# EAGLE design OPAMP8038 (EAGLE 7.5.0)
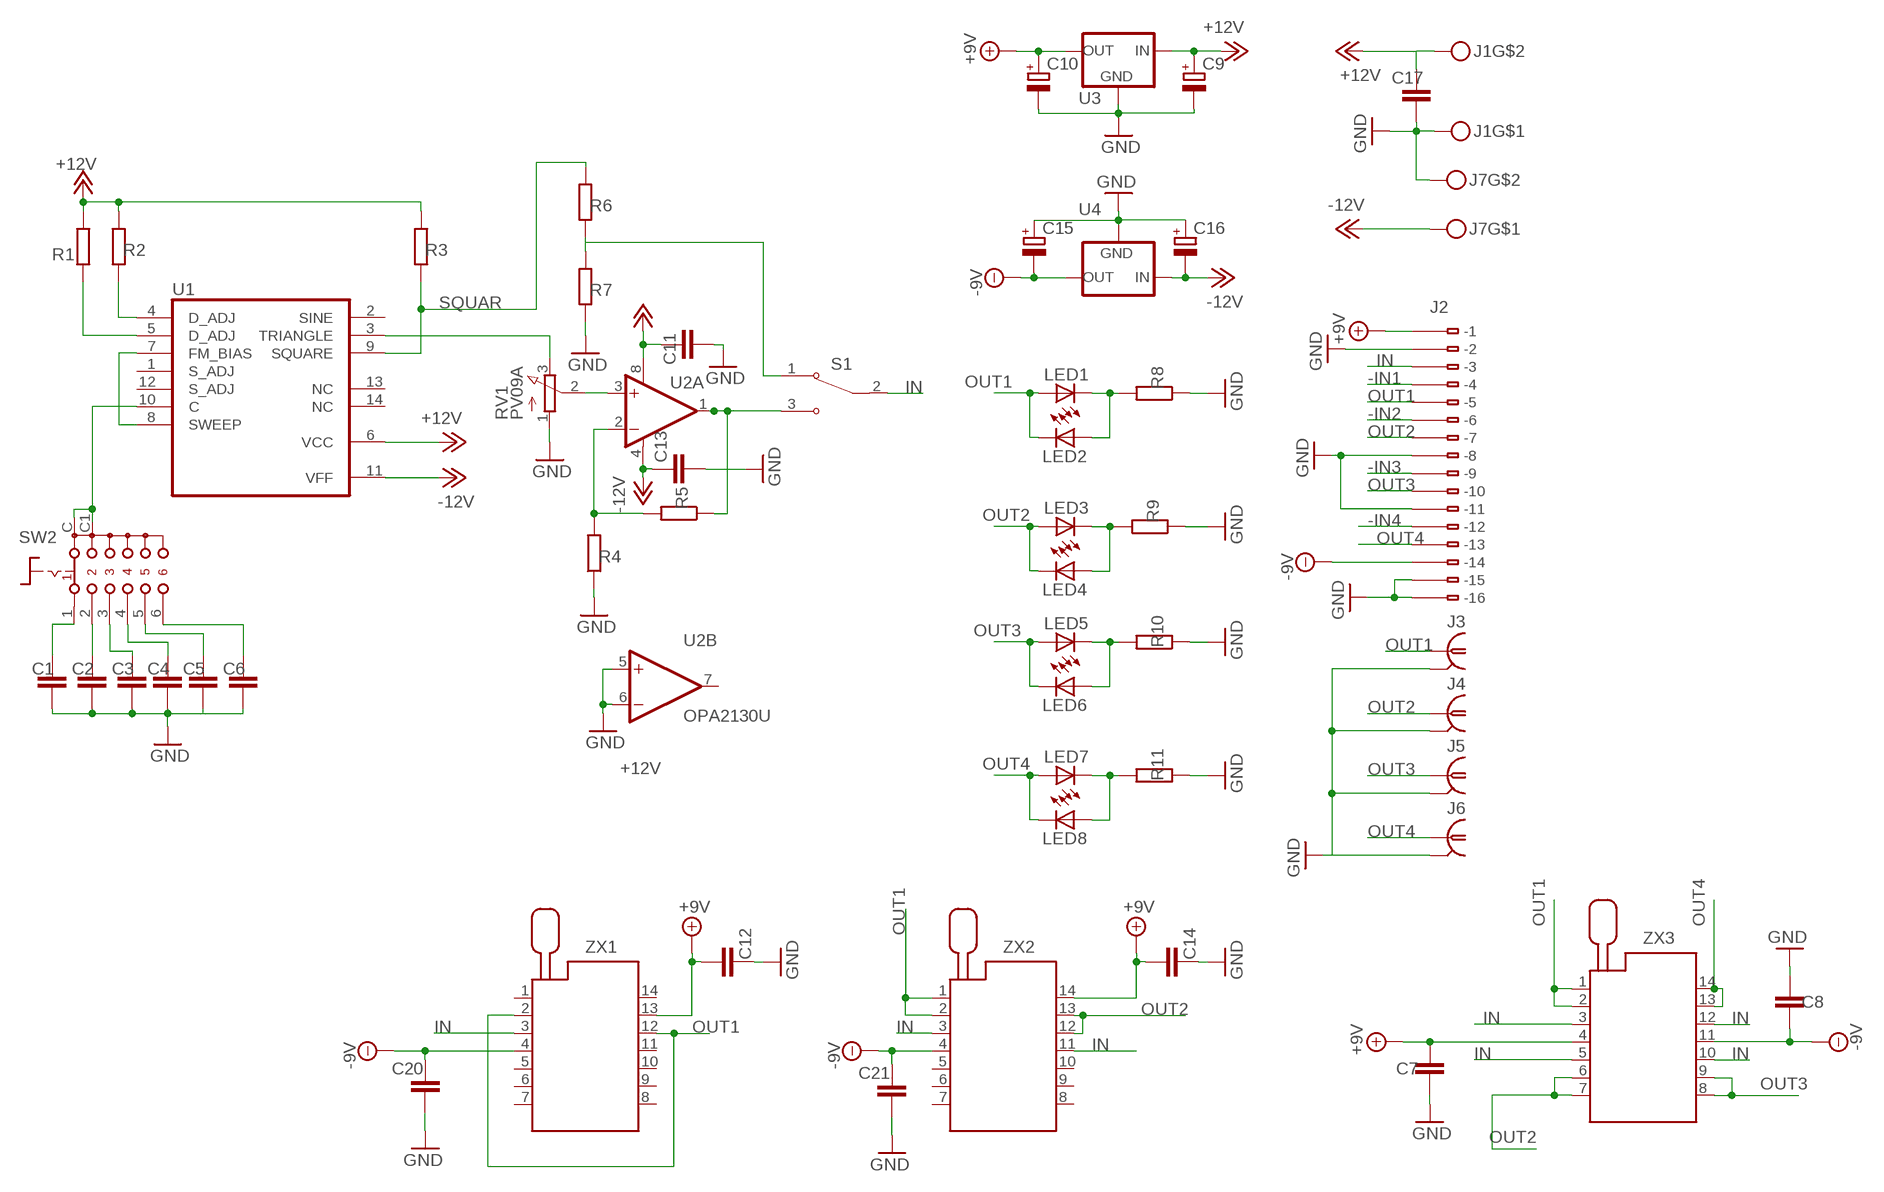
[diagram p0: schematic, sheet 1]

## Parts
C1  C-EUC1206  [C1206]
C2  C-EUC1206  [C1206]
C3  C-EUC1206  [C1206]
C4  C-EUC1206  [C1206]
C5  C-EUC1206  [C1206]
C6  C-EUC1206  [C1206]
C7  C-EUC1206  [C1206]
C8  C-EUC1206  [C1206]
C9  CPOL-EUSMCC  [SMC_C]
C10  CPOL-EUSMCC  [SMC_C]
C11  C-EUC1206  [C1206]
C12  C-EUC1206  [C1206]
C13  C-EUC1206  [C1206]
C14  C-EUC1206  [C1206]
C15  CPOL-EUSMCC  [SMC_C]
C16  CPOL-EUSMCC  [SMC_C]
C17  C-EUC1206  [C1206]
C20  C-EUC1206  [C1206]
C21  C-EUC1206  [C1206]
J1  MKDSN1,5-2-5,08  [MKDSN1,5-2-5,08]
J2  233-116  [233-116]
J3  1-227161-0  [AMP_227161]
J4  1-227161-0  [AMP_227161]
J5  1-227161-0  [AMP_227161]
J6  1-227161-0  [AMP_227161]
J7  MKDSN1,5-2-5,08  [MKDSN1,5-2-5,08]
LED1  LED5MM  [LED5MM]
LED2  LED5MM  [LED5MM]
LED3  LED5MM  [LED5MM]
LED4  LED5MM  [LED5MM]
LED5  LED5MM  [LED5MM]
LED6  LED5MM  [LED5MM]
LED7  LED5MM  [LED5MM]
LED8  LED5MM  [LED5MM]
R1  R-EU_R1206  [R1206]
R2  R-EU_R1206  [R1206]
R3  R-EU_R1206  [R1206]
R4  R-EU_R1206  [R1206]
R5  R-EU_R1206  [R1206]
R6  R-EU_R1206  [R1206]
R7  R-EU_R1206  [R1206]
R8  R-EU_R1206  [R1206]
R9  R-EU_R1206  [R1206]
R10  R-EU_R1206  [R1206]
R11  R-EU_R1206  [R1206]
RV1  PV09A  [PTV09]
S1  100SP1T6B11M1QE  [SW_100SP1T6B11M1QE]
SW2  SS-10-16  [SS-10-16]
U1  XR-8038  [DIL14]
U2  OPA2130U  [SO08]
U3  78XXL  [78XXL]
U4  79XXL  [79XXL]
ZX1  214-3339-00-0602J  [214-3339-00-0602J]
ZX2  214-3339-00-0602J  [214-3339-00-0602J]
ZX3  214-3339-00-0602J  [214-3339-00-0602J]

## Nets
+9V: C7.1 C10.+ C12.2 C14.2 J2.B1(B-1) U3.OUT ZX1.13 ZX2.14 ZX3.4
+12V: C9.+ C11.1 C17.1 J1.2 R1.2 R2.2 R3.2 U1.6(VCC) U2.8(A:V+) U3.IN
-9V: C8.1 C15.- C20.1 C21.1 J2.B14(B-14) U4.OUT ZX1.4 ZX2.4 ZX3.11
-12V: C13.1 C16.- J7.1 U1.11(VFF) U2.4(A:V-) U4.IN
-IN1: J2.B4(B-4)
-IN2: J2.B6(B-6)
-IN3: J2.B9(B-9)
-IN4: J2.B12(B-12)
GND: C1.2 C2.2 C3.2 C4.2 C5.2 C6.2 C7.2 C8.2 C9.- C10.- C11.2 C12.1 C13.2 C14.1 C15.+ C16.+ C17.2 C20.2 C21.2 J1.1 J2.B2(B-2) J2.B8(B-8) J2.B11(B-11) J2.B15(B-15) J2.B16(B-16) J3.2 J4.2 J5.2 J6.2 J7.2 R4.1 R7.1 R8.1 R9.1 R10.1 R11.1 RV1.1(A) U2.5(B:+IN) U2.6(B:-IN) U3.GND U4.GND
IN: J2.B3(B-3) S1.2 ZX1.3 ZX2.3 ZX2.11 ZX3.3 ZX3.5 ZX3.10 ZX3.12
N$1: R6.1 R7.2 S1.1
N$2: C6.1 SW2.6
N$3: R2.1 U1.4(D_ADJ)
N$4: R1.1 U1.5(D_ADJ)
N$5: RV1.2(S) U2.3(A:+IN)
N$6: RV1.3(E) U1.3(TRIANGLE)
N$7: R4.2 R5.2 U2.2(A:-IN)
N$8: R5.1 S1.3 U2.1(A:OUT)
N$9: U1.7(FM_BIAS) U1.8(SWEEP)
N$10: SW2.C SW2.C1 U1.10(C)
N$11: LED1.K(C) LED2.A R8.2
N$12: C1.1 SW2.1
N$13: C2.1 SW2.2
N$14: C3.1 SW2.3
N$15: C4.1 SW2.4
N$16: C5.1 SW2.5
N$18: LED3.K(C) LED4.A R9.2
N$20: LED5.K(C) LED6.A R10.2
N$23: LED7.K(C) LED8.A R11.2
OUT1: J2.B5(B-5) J3.1 LED1.A LED2.K(C) ZX1.2 ZX1.12 ZX2.1 ZX2.2 ZX3.1 ZX3.2
OUT2: J2.B7(B-7) J4.1 LED3.A LED4.K(C) ZX2.12 ZX2.13 ZX3.6 ZX3.7
OUT3: J2.B10(B-10) J5.1 LED5.A LED6.K(C) ZX3.8 ZX3.9
OUT4: J2.B13(B-13) J6.1 LED7.A LED8.K(C) ZX3.13 ZX3.14
SQUAR: R3.1 R6.2 U1.9(SQUARE)
Unconnected: J2.A1(-1) J2.A2(-2) J2.A3(-3) J2.A4(-4) J2.A5(-5) J2.A6(-6) J2.A7(-7) J2.A8(-8) J2.A9(-9) J2.A10(-10) J2.A11(-11) J2.A12(-12) J2.A13(-13) J2.A14(-14) J2.A15(-15) J2.A16(-16) U1.1(S_ADJ) U1.2(SINE) U1.12(S_ADJ) U1.13(NC) U1.14(NC) U2.7(B:OUT) ZX1.1 ZX1.5 ZX1.6 ZX1.7 ZX1.8 ZX1.9 ZX1.10 ZX1.11 ZX1.14 ZX2.5 ZX2.6 ZX2.7 ZX2.8 ZX2.9 ZX2.10

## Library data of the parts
C1-C8 C11-C14 C17 C20 C21 = rcl:C-EU: CAPACITOR, European symbol
C9 C10 C15 C16 = rcl:CPOL-EU: POLARIZED CAPACITOR, European symbol
J1 J7 = con-phoenix-508:MKDSN1,5-2-5,08
J2 = con-wago:233-116: WAGO Cage Clamp; MPN: 233-116; OC_FARNELL: unknown; OC_NEWARK: 28K9054
J3-J6 = con-coax:?227161*: JACK, RIGHT ANGLE, 50 OHM, PCB, BNC; MF: TYCO ELECTRONICS; MPN: 1-227161; OC_FARNELL: unknown; OC_NEWARK: 33B3200
LED1-LED8 = led:LED: LED
R1-R11 = rcl:R-EU_: RESISTOR, European symbol
RV1 = pot:PV09A
S1 = 100SP1T6B11M1QE:100SP1T6B11M1QE: Check availability; AVAILABILITY: Not in stock; CHECK_PRICES: https://www.snapeda.com/parts/100SP1T6B11M1QE/E-Switch/view-part/?ref=eda; DESCRIPTION: Toggle Switches TOGGLE, SPDT , On-On, Panel Mount; MF: E-Switch; MP: 100SP1T6B11M1QE; PACKAGE: None; PRICE: None; SNAPEDA_LINK: https://www.snapeda.com/parts/100SP1T6B11M1QE/E-Switch/view-part/?ref=snap
SW2 = switch:SS-10-16: Rotary Switch, Through Hole, 6 Position, 1 Pole
U1 = exar:XR-8038: Precision WAVEFORM GENERATOR; OC_FARNELL: unknown; OC_NEWARK: unknown
U2 = burr-brown:OPA2130: Operational Amplifier; MF: TEXAS INSTRUMENTS; MPN: OPA2130UA; OC_FARNELL: 1459554; OC_NEWARK: 35C1841
U3 = v-reg:78XXL: VOLTAGE REGULATOR
U4 = v-reg:79XXL: VOLTAGE REGULATOR
ZX1-ZX3 = con-3m:214-3339-00-0602J: Zero Insertion Force Socked Source: http://www.3M.com/ehpd; MF: 3M; MPN: 214-3339-00-0602J; OC_FARNELL: 1247151; OC_NEWARK: 85K7793

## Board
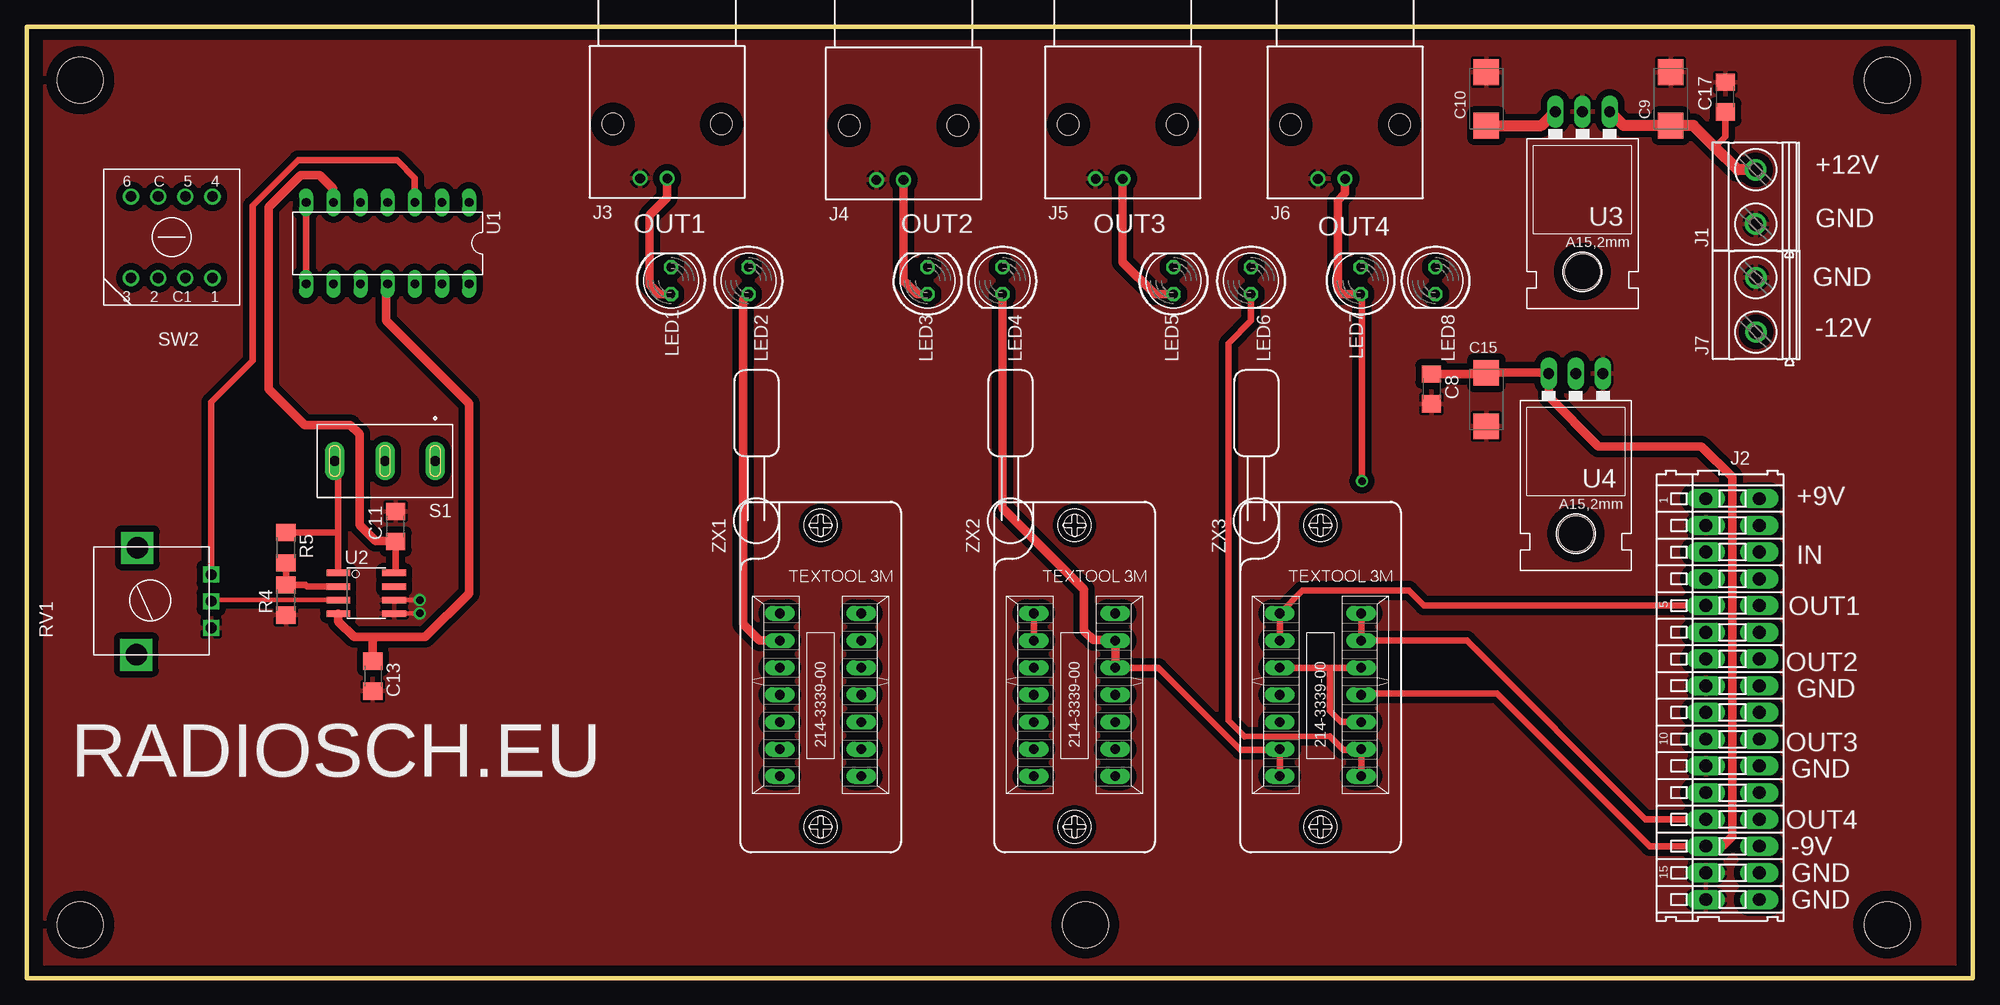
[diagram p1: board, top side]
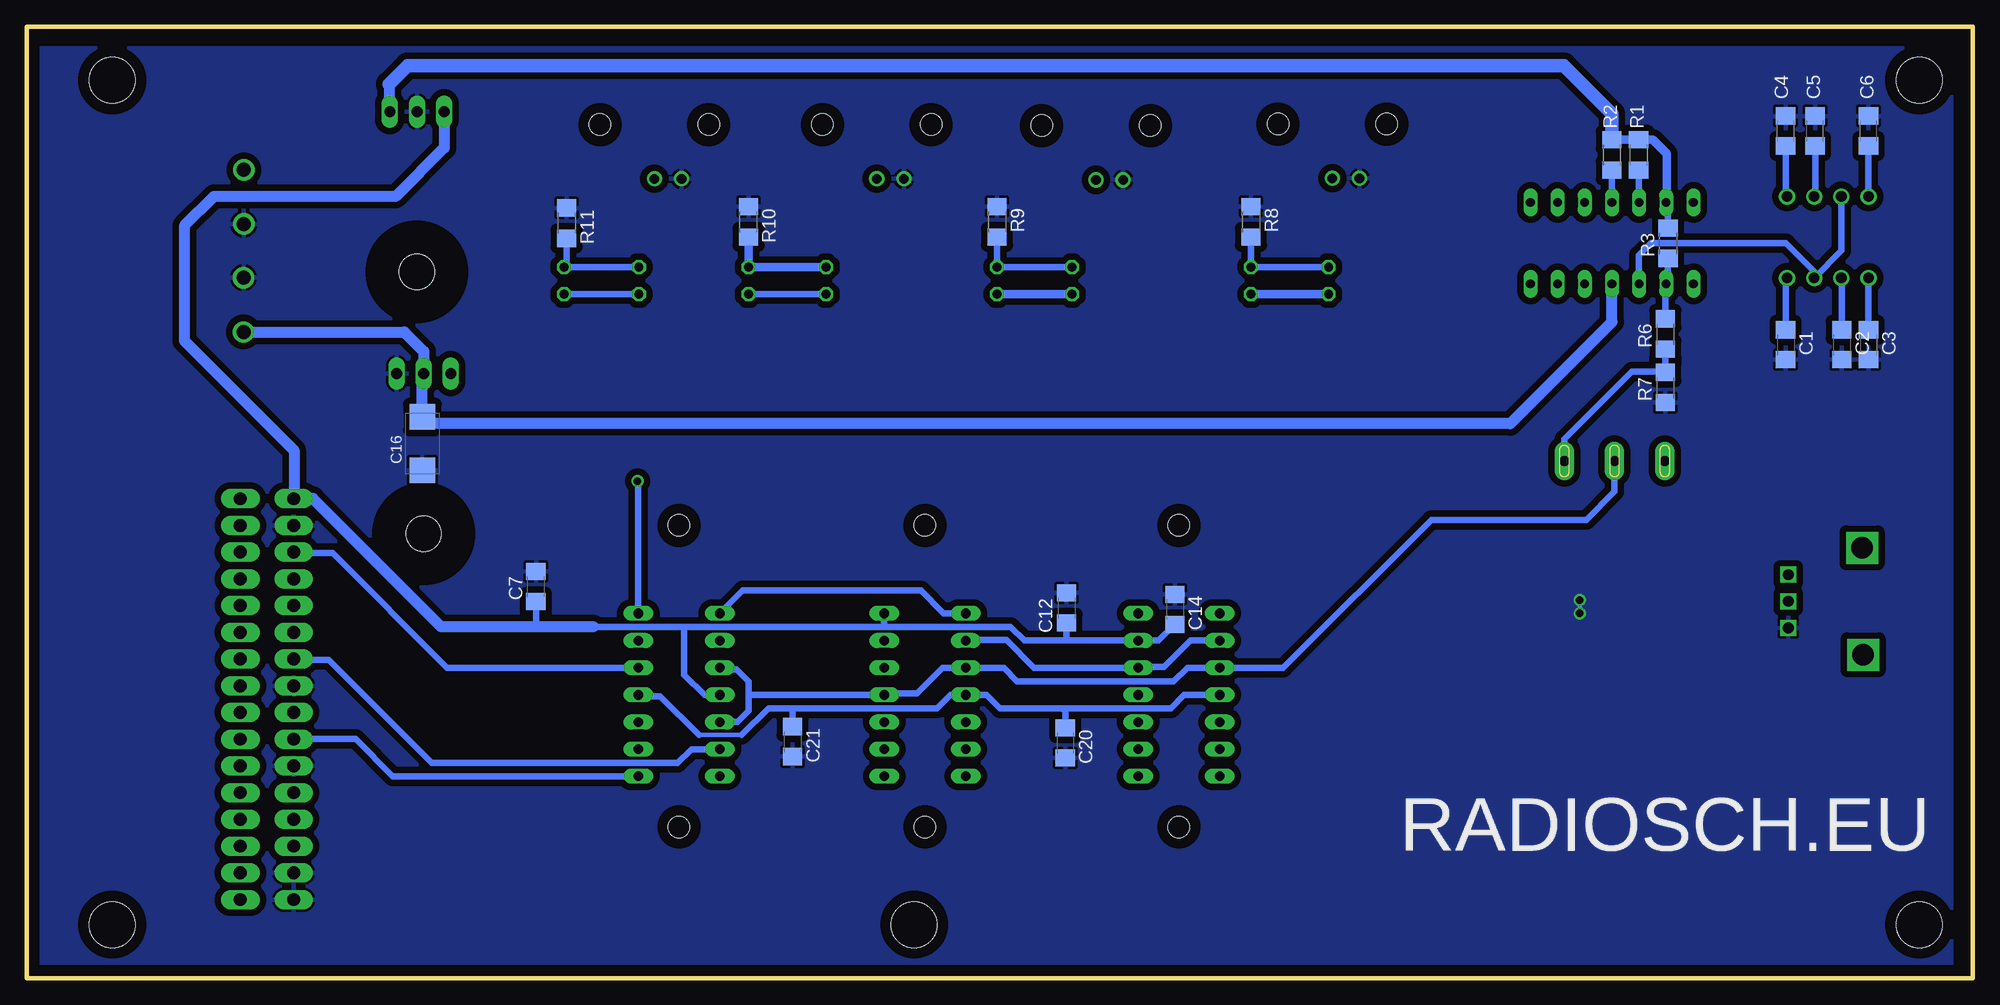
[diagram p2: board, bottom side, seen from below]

Size 182 x 89 mm. Coordinates in mm from the lower left corner, seen from the top.
Outline: 0,0 182,0 182,89 0,89 0,0
Copper layers (1*16): Top 0.035mm / dielectric 1.5mm / Bottom 0.035mm
Design rules "default": minimum track width 10mil, minimum drill 24mil, track to track 8mil, track to pad 8mil, pad to pad 8mil, via to via 8mil, smd to smd 8mil, copper to edge 40mil, drill to drill 8mil, minimum pad ring 10mil, minimum via ring 8mil, stop-mask expansion 4mil, vias tented up to drill 0mil, thermal gap 10mil
Holes 4.3 mm at 5,84 5,5 99,5 174,5 174,84

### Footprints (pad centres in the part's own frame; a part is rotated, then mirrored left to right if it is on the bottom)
C1206 = smd 1.6 x 1.8: 1 -1.4,0; 2 1.4,0
SMC_C = smd 2.4 x 2.4: + -2.5,0; - 2.5,0
MKDSN1,5-2-5,08 = drill 1.3 pad 2: 1 -2.561,0.025; 2 2.519,0.025
233-116 = drill 1.2 long: A1 -18.75,2.5; A2 -16.25,2.5; A3 -13.75,2.5; A4 -11.25,2.5; A5 -8.75,2.5; A6 -6.25,2.5; A7 -3.75,2.5; A8 -1.25,2.5; A9 1.25,2.5; A10 3.75,2.5; A11 6.25,2.5; A12 8.75,2.5; A13 11.25,2.5; A14 13.75,2.5; A15 16.25,2.5; A16 18.75,2.5; B1 -18.75,-2.5; B2 -16.25,-2.5; B3 -13.75,-2.5; B4 -11.25,-2.5; B5 -8.75,-2.5; B6 -6.25,-2.5; B7 -3.75,-2.5; B8 -1.25,-2.5; B9 1.25,-2.5; B10 3.75,-2.5; B11 6.25,-2.5; B12 8.75,-2.5; B13 11.25,-2.5; B14 13.75,-2.5; B15 16.25,-2.5; B16 18.75,-2.5
AMP_227161 = drill 0.9 pad 1.27: 1 0,-5.08; 2 -2.54,-5.08 | hole 2: -5.08,0; 5.08,0
LED5MM = drill 0.813 octagon: A -1.27,0; K 1.27,0
R1206 = smd 1.6 x 1.803: 1 -1.422,0; 2 1.422,0
PTV09 = drill 1 square: 1 -2.5,0; 2 0,0; 3 2.5,0 | drill 2 square: P$4 -5,7; P$5 5,6.9
SW_100SP1T6B11M1QE = drill 0.91 pad 1.81 long: 1 -4.7,0; 2 0,0; 3 4.7,0
SS-10-16 = drill 1: 1 -7.62,0; 2 -2.54,0; 3 0,0; 4 -7.62,-7.62; 5 -5.08,-7.62; 6 0,-7.62; C -2.54,-7.62; C1 -5.08,0
DIL14 = drill 0.813 long: 1 -7.62,-3.81; 2 -5.08,-3.81; 3 -2.54,-3.81; 4 0,-3.81; 5 2.54,-3.81; 6 5.08,-3.81; 7 7.62,-3.81; 8 7.62,3.81; 9 5.08,3.81; 10 2.54,3.81; 11 0,3.81; 12 -2.54,3.81; 13 -5.08,3.81; 14 -7.62,3.81
SO08 = smd 0.61 x 2.21: 1 -1.905,-2.616; 2 -0.635,-2.616; 3 0.635,-2.616; 4 1.905,-2.616; 5 1.905,2.616; 6 0.635,2.616; 7 -0.635,2.616; 8 -1.905,2.616
78XXL = drill 1.016 long: GND 0,-3.81; IN -2.54,-3.81; OUT 2.54,-3.81 | hole 3.302: 0,11.176
79XXL = drill 1.016 long: GND -2.54,-3.81; IN 0,-3.81; OUT 2.54,-3.81 | hole 3.302: 0,11.176
214-3339-00-0602J = drill 0.9 long: 1 -7.62,-3.81; 2 -5.08,-3.81; 3 -2.54,-3.81; 4 0,-3.81; 5 2.54,-3.81; 6 5.08,-3.81; 7 7.62,-3.81; 8 7.62,3.81; 9 5.08,3.81; 10 2.54,3.81; 11 0,3.81; 12 -2.54,3.81; 13 -5.08,3.81; 14 -7.62,3.81 | hole 2: 12.35,0; -15.85,0

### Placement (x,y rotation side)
C1  17.5,59.25 270 bottom
C2  12.25,59.25 270 bottom
C3  9.75,59.25 270 bottom
C4  17.5,79.25 90 bottom
C5  14.75,79.25 90 bottom
C6  9.75,79.25 90 bottom
C7  134.38,36.62 90 bottom
C8  131.38,55.12 270 top
C9  153.75,82.25 90 top
C10  136.5,82.25 90 top
C11  34.5,42.25 90 top
C12  84.75,34.62 270 bottom
C13  32.38,28.25 270 top
C14  74.62,34.5 270 bottom
C15  136.5,54.12 90 top
C16  145,50 90 bottom
C17  158.85,82.42 90 top
C20  84.88,22 270 bottom
C21  110.38,22.12 270 bottom
J1  161.72,73.1 90 top
J2  159.53,26.1 270 top
J3  59.9,79.9 0 top
J4  82,79.75 0 top
J5  102.5,79.85 0 top
J6  123.3,79.85 0 top
J7  161.75,63 90 top
LED1  60.25,65.25 90 top
LED2  67.5,65.25 270 top
LED3  84.25,65.25 90 top
LED4  91.25,65.25 270 top
LED5  107.25,65.25 90 top
LED6  114.5,65.25 270 top
LED7  124.75,65.25 90 top
LED8  131.75,65.25 270 top
R1  31.25,77 90 bottom
R2  33.75,77 90 bottom
R3  28.5,68.75 90 bottom
R4  24.25,35.38 90 top
R5  24.25,40.25 270 top
R6  28.75,60.25 90 bottom
R7  28.75,55.25 90 bottom
R8  67.5,70.75 270 bottom
R9  91.25,70.75 270 bottom
R10  114.5,70.75 270 bottom
R11  131.5,70.62 270 bottom
RV1  17.25,35.25 90 top
S1  33.5,48.38 180 top
SW2  9.75,65.5 180 top
U1  33.75,68.75 180 top
U2  31.75,36 270 top
U3  145.5,77.25 180 top
U4  144.88,52.75 180 top
ZX1  74.25,26.5 270 top
ZX2  98,26.5 270 top
ZX3  121,26.5 270 top

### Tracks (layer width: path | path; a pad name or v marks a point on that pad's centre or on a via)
+9V
  Top 1.016: C10.+ 141.65,79.75 U3.OUT
  Bottom 0.61: 84.88,31.58 ZX1.13 76.14,31.58 C14.2 | 84.88,31.58 88.7,31.58 90,32.88 101.88,32.88 | 101.88,32.88 120.62,32.88 | 120.62,32.88 129,32.88 | C12.2 84.75,31.7 84.88,31.58 | ZX2.14 101.81,32.94 101.88,32.88 | ZX3.4 118.62,26.5 120.5,28.38 120.5,32.75 120.62,32.88 | C7.1 134.38,33 134.25,32.88
  Bottom 1.016: 129,32.88 134.25,32.88 143.25,32.88 155.25,44.88 157,44.88 | U3.OUT 142.96,77.67 147.5,73.12 164.5,73.12 167.25,70.38 167.25,59.62 157,49.38 157,44.88 | 157,44.88 J2.B1
+12V
  Top 0.61: C11.1 34.5,38.04 U2.8 | C17.1 158.85,78.72 157.88,77.75
  Top 0.813: U1.6 28.67,73.83 27.38,75.12 25.62,75.12 22.62,72.12 22.62,55.12 26,51.75 30.25,51.75 31.12,50.88 31.12,42.38 32.62,40.88 34.48,40.88 C11.1
  Top 1.016: J1.2 160.01,75.62 157.88,77.75 155.88,79.75 C9.+ 149.35,79.75 U3.IN
  Bottom 0.61: R3.2 28.5,72.39 U1.6
  Bottom 0.813: U1.6 28.62,72.61 28.62,77.12 29.92,78.42 R1.2 R2.2
  Bottom 1.016: U3.IN 148.04,83.54 148.12,83.62
  Bottom 1.27: R2.2 33.75,80.88 38.25,85.38 146.38,85.38 148.12,83.62
-9V
  Top 0.61: J2.B14 151.78,12.35 137.5,26.62 124.94,26.62 ZX3.11
  Top 0.813: J2.B14 157.05,12.38 158.62,12.38 159.5,13.25 159.5,46.88 156.62,49.75 147,49.75 142.34,54.41 U4.OUT 142.27,56.62 C15.- 136.4,56.52 C8.1
  Bottom 0.406: 115.12,22.75 119.12,22.75
  Bottom 0.61: ZX1.4 73.75,26.5 75,25.25 85.12,25.25 | 85.12,25.25 91,25.25 92.25,26.5 ZX2.4 95.62,26.5 96.88,25.25 110.25,25.25 | 110.25,25.25 112.62,25.25 115.12,22.75 | 119.12,22.75 122.75,26.38 124.69,26.38 ZX3.11 | C21.1 110.38,25.12 110.25,25.25 | C20.1 84.88,25 85.12,25.25
-12V
  Top 0.813: U1.11 33.62,64.81 33.62,61.5 41.38,53.75 41.38,36 37.27,31.9 32.62,31.9 | 32.62,31.9 30.6,31.9 29.12,33.38 U2.4 | C13.1 32.38,31.65 32.62,31.9
  Bottom 1.016: U1.11 33.75,61.38 43.25,51.88 144.38,51.88 C16.- 145,56.44 U4.IN 144.88,58.62 146.69,60.44 J7.1
GND  (via drill 0.7)
  Top 0.406: U2.5 36.72,34.09 v36.75,34.12 | v36.75,35.38 U2.6
  Bottom 0.406: v36.75,34.12 v36.75,35.38
  pour Bottom (isolate 0.61): 2,87 186,87 186,1 2,1
  pour Top (isolate 0.61): 1.75,87.75 180.25,87.75 180.25,1.25 1.75,1.25
IN
  Top 0.61: ZX3.3 121.62,29.04 | 121.62,29.04 ZX3.12 | ZX3.10 122.92,23.96 121.88,25 121.88,28.79 121.62,29.04
  Bottom 0.61: ZX3.3 117.03,28.88 115.62,28.88 114.5,27.75 114.5,26.38 | 114.5,26.38 114.5,25 115.54,23.96 ZX3.5 | 114.5,26.38 114.38,26.5 ZX2.11 101.69,26.62 98.75,26.62 96.33,29.04 ZX2.3 94.15,29 90.62,29 89.38,27.75 74.75,27.75 73.46,29.04 ZX1.3 70.4,29 64.5,29 50.62,42.88 36.12,42.88 33.5,45.5 S1.2 | ZX3.12 142.66,29.04 153.38,39.75 156.38,39.75 156.5,39.62 156.8,39.62 J2.B3
N$1
  Bottom 0.61: S1.1 38.2,50.42 31.88,56.75 28.83,56.75 R7.2 R6.1
N$2
  Bottom 0.61: C6.1 SW2.6
N$3
  Bottom 0.61: U1.4 R2.1
N$4
  Bottom 0.61: U1.5 31.21,75.54 R1.1
N$5
  Top 0.406: U2.3 17.36,35.37 RV1.2
N$6
  Top 0.61: RV1.3 17.25,53.88 21.12,57.75 21.12,72.25 25.38,76.5 34.62,76.5 36.29,74.83 U1.3
N$7
  Top 0.61: R5.2 R4.2 26.08,36.8 26.25,36.62 U2.2
N$8
  Top 0.61: U2.1 29.13,41.75 | 29.13,41.75 29.13,48.04 S1.3 | R5.1 29.06,41.67 29.13,41.75
N$9
  Top 0.61: U1.8 U1.7
N$10
  Bottom 0.61: U1.10 31.25,64.98 31.25,67.62 30.12,68.75 17.5,68.75 14.83,66.08 SW2.C1 12.29,68.04 SW2.C
N$11
  Bottom 0.61: LED1.K LED2.A R8.2
N$12
  Bottom 0.61: C1.1 17.5,65.37 SW2.1
N$13
  Bottom 0.61: C2.1 12.25,65.46 SW2.2
N$14
  Bottom 0.61: C3.1 SW2.3
N$15
  Bottom 0.61: C4.1 17.5,73.25 SW2.4
N$16
  Bottom 0.61: C5.1 14.75,73.2 SW2.5
N$18
  Bottom 0.61: LED3.K 90.75,66.52 | 90.75,66.52 LED4.A | R9.2 91.25,67.02 90.75,66.52
N$20
  Bottom 0.813: R10.2 LED6.A LED5.K
N$23
  Bottom 0.61: R11.2 131.5,66.77 LED8.A LED7.K
OUT1
  Top 0.61: ZX2.2 ZX2.1 | ZX3.2 ZX3.1 119.32,36.25 129.25,36.25 130.65,34.85 J2.B5
  Top 0.813: J3.1 59.9,73.03 58.25,71.38 58.25,64.88 59.12,64 60.23,64 LED1.A | ZX1.2 68.55,31.58 67,33.12 67,63.48 LED2.K
  Bottom 0.61: ZX1.2 73.17,31.58 75.62,29.12 77.97,29.12 ZX1.12 87.79,29.04 90.38,31.62 94.14,31.62 ZX2.2 | ZX2.1 96.25,34.12 98.38,36.25 115.06,36.25 ZX3.1
  Bottom 0.813: LED2.K LED1.A
OUT2
  Top 0.61: ZX2.12 105.83,29.04 113.5,21.38 117.14,21.38 ZX3.6 ZX3.7
  Top 0.813: LED4.K 91.25,44 98.88,36.38 98.88,32.5 99.75,31.62 101.25,31.62 | 101.25,31.62 101.77,31.62 ZX2.13 | ZX2.12 101.81,31.07 101.25,31.62 | J4.1 82,65.25 83.25,64 84.23,64 LED3.A
  Bottom 0.61: ZX3.6 119.83,21.42 121.12,20.12 144.12,20.12 153.75,29.75 156.93,29.75 J2.B7
  Bottom 0.813: LED3.A LED4.K
OUT3
  Top 0.5: 113.88,22.62 121.88,22.62
  Top 0.61: ZX3.8 ZX3.9 124.77,21.38 123.12,21.38 121.88,22.62 | LED6.K 114.5,61.5 112.38,59.38 112.38,24.12 113.88,22.62
  Top 0.813: J5.1 102.5,67 105.5,64 107.23,64 LED5.A
  Bottom 0.61: ZX3.8 147.75,18.88 151.25,22.38 157,22.38 J2.B10 | LED5.A LED6.K
OUT4  (via drill 0.7)
  Top 0.61: J2.B13 157,14.88 151.38,14.88 134.67,31.58 ZX3.13 ZX3.14 | v124.88,46.5 124.88,63.85 LED7.A
  Top 0.813: J6.1 123.3,73.42 122.62,72.75 122.62,64.38 123,64 124.73,64 LED7.A
  Bottom 0.61: ZX3.14 124.81,46.44 v124.88,46.5 | LED8.K LED7.A
SQUAR
  Top 0.61: 28.75,64.86 U1.9
  Bottom 0.61: R3.1 28.5,65.11 U1.9 28.75,64.86 R6.2

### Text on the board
tPlace: +12V | OUT1 | OUT2 | OUT3 | OUT4 | GND | GND | -12V | +9V | IN | OUT1 | OUT2 | GND | RADIOSCH.EU | OUT3 | GND | OUT4 | -9V | GND | GND
bPlace: RADIOSCH.EU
